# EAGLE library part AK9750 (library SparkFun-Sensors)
AK9750/AK9753 Human Movement Sensor
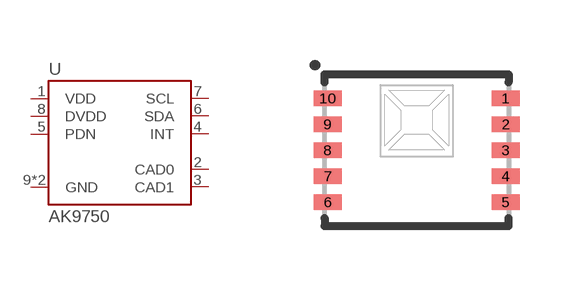
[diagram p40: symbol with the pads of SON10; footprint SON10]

Designator prefix U

## AK9750 (PROD_ID: SEN-13737; VALUE: AK9750)  [SON10]
1  VDD
2  CAD0
3  CAD1
4  INT
5  PDN
6  SDA
7  SCL
8  DVDD
9  GND
10  GND

## AK9750" (PROD_ID: SEN_13772; VALUE: AK9753)  [SON10]
1  GND
2  GND
3  DVDD
4  SCL
5  SDA
6  PDN
7  INT
8  CAD1
9  CAD0
10  VDD

## Footprint SON10 (pad centres in mm)
smd 0.7 x 0.38: 1 2.225,1.3; 2 2.225,0.65; 3 2.225,0; 4 2.225,-0.65; 5 2.225,-1.3; 6 -2.225,-1.3; 7 -2.225,-0.65; 8 -2.225,0; 9 -2.225,0.65; 10 -2.225,1.3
